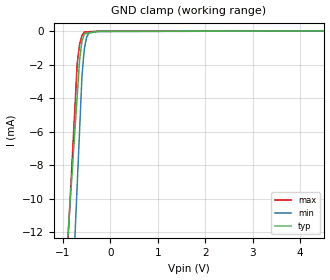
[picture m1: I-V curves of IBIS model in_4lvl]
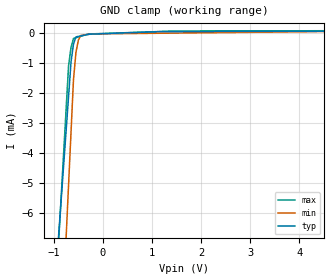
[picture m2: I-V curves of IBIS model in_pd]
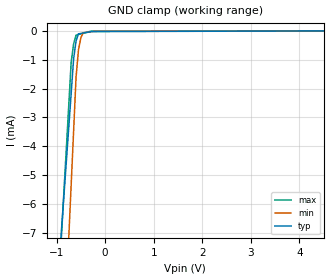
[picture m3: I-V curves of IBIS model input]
[IBIS Ver]   3.2
[Comment Char] |_char
[File Name]   pcm3168tpap.ibs
[File Rev]   3.0
[Source]
| This model file was created by Teraspeed Consulting Group LLC
| (http://www.teraspeed.com/).
[Date]   05-08-2008
[Notes]   Quality Check of this IBIS model: Model Passes IBIS Check
   Model parses into ICX IS. Simulation done with Hyperlynx.
   1. MIN TYP MAX information is based on Temprature and Voltage
   characteristics only.
[Disclaimer]
| This model is designed as an aid for customers of Texas Instruments.
| TI and its licensors and suppliers make no warranties, either expressed
| or implied, with respect to this  model, including the warranties of
| merchantability or fitness for a particular purpose.
| The model is provided solely on an "as is" basis. The entire risk as to
| its quality and performance is with the customer.
[Copyright]
| (C) Copyright 2008 Texas Instruments Incorporated. All rights reserved.
[Component]   PCM3168TPAP
[Manufacturer] TI
[Package]
| variable   typ   min   max
R_pkg  6.05E-02  5.80E-02  6.50E-02
L_pkg  5.05E-09  4.85E-09  5.38E-09
C_pkg  2.68E-13  2.40E-13  3.00E-13
[Pin] signal_name  model_name  R_pin  L_pin C_pin
1   VCOMAD   term   6.50E-02  5.38E-09  3.00E-13
2   AGNDAD2   GND   6.30E-02  5.25E-09  2.90E-13
3   VCCAAD2   POWER   6.20E-02  5.13E-09  2.80E-13
4   RST   in_pd   6.00E-02  5.04E-09  2.70E-13
5   OVF   output  5.90E-02  4.95E-09  2.60E-13
6   LRCKAD   io_pd   5.90E-02  4.90E-09  2.50E-13
7   BCKAD   io_pd   5.80E-02  4.87E-09  2.50E-13
8   DOUT1   output  5.80E-02  4.85E-09  2.40E-13
9   DOUT2   output  5.80E-02  4.85E-09  2.40E-13
10   DOUT3   output  5.80E-02  4.87E-09  2.50E-13
11   DGND2   GND   5.90E-02  4.90E-09  2.50E-13
12   VDD2   POWER   5.90E-02  4.95E-09  2.60E-13
13   ZERO   output  6.00E-02  5.04E-09  2.70E-13
14   VCCDA1   POWER   6.20E-02  5.13E-09  2.80E-13
15   VCOMDA   term   6.30E-02  5.25E-09  2.90E-13
16   AGNDDA1   GND   6.50E-02  5.38E-09  3.00E-13
17   VOUT8+   term   6.50E-02  5.38E-09  3.00E-13
18   VOUT8-   term   6.30E-02  5.25E-09  2.90E-13
19   VOUT7+   term   6.20E-02  5.13E-09  2.80E-13
20   VOUT7-   term   6.00E-02  5.04E-09  2.70E-13
21   VOUT6+   term   5.90E-02  4.95E-09  2.60E-13
22   VOUT6-   term   5.90E-02  4.90E-09  2.50E-13
23   VOUT5+   term   5.80E-02  4.87E-09  2.50E-13
24   VOUT5-   term   5.80E-02  4.85E-09  2.40E-13
25   VOUT4+   term   5.80E-02  4.85E-09  2.40E-13
26   VOUT4-   term   5.80E-02  4.87E-09  2.50E-13
27   VOUT3+   term   5.90E-02  4.90E-09  2.50E-13
28   VOUT3-   term   5.90E-02  4.95E-09  2.60E-13
29   VOUT2+   term   6.00E-02  5.04E-09  2.70E-13
30   VOUT2-   term   6.20E-02  5.13E-09  2.80E-13
31   VOUT1+   term   6.30E-02  5.25E-09  2.90E-13
32   VOUT1-   term   6.50E-02  5.38E-09  3.00E-13
33   AGNDDA2   GND   6.50E-02  5.38E-09  3.00E-13
34   VCCDA2   POWER   6.30E-02  5.25E-09  2.90E-13
35   LRCKDA   io_pd   6.20E-02  5.13E-09  2.80E-13
36   BCKDA   io_pd   6.00E-02  5.04E-09  2.70E-13
37   DIN1   input   5.90E-02  4.95E-09  2.60E-13
38   DIN2   input   5.90E-02  4.90E-09  2.50E-13
39   DIN3   input   5.80E-02  4.87E-09  2.50E-13
40   DIN4   input   5.80E-02  4.85E-09  2.40E-13
41   SCKI   input   5.80E-02  4.85E-09  2.40E-13
42   MC/SCL/FMT   input   5.80E-02  4.87E-09  2.50E-13
43   MDI/SDA/DEMP io_od   5.90E-02  4.90E-09  2.50E-13
44   MDO/ADR1/MD1 io   5.90E-02  4.95E-09  2.60E-13
45   MS/ADR0/MD0  in_pd   6.00E-02  5.04E-09  2.70E-13
46   VDD1   POWER   6.20E-02  5.13E-09  2.80E-13
47   DGND1   GND   6.30E-02  5.25E-09  2.90E-13
48   MODE   in_4lvl 6.50E-02  5.38E-09  3.00E-13
49   VCCAD1   POWER   6.50E-02  5.38E-09  3.00E-13
50   AGNDAD1   GND   6.30E-02  5.25E-09  2.90E-13
51   VIN1-   term   6.20E-02  5.13E-09  2.80E-13
52   VIN1+   term   6.00E-02  5.04E-09  2.70E-13
53   VIN2-   term   5.90E-02  4.95E-09  2.60E-13
54   VIN2+   term   5.90E-02  4.90E-09  2.50E-13
55   VIN3-   term   5.80E-02  4.87E-09  2.50E-13
56   VIN3+   term   5.80E-02  4.85E-09  2.40E-13
57   VIN4-   term   5.80E-02  4.85E-09  2.40E-13
58   VIN4+   term   5.80E-02  4.87E-09  2.50E-13
59   VREFAD1   term   5.90E-02  4.90E-09  2.50E-13
60   VREFAD2   term   5.90E-02  4.95E-09  2.60E-13
61   VIN5-   term   6.00E-02  5.04E-09  2.70E-13
62   VIN5+   term   6.20E-02  5.13E-09  2.80E-13
63   VIN6-   term   6.30E-02  5.25E-09  2.90E-13
64   VIN6+   term   6.50E-02  5.38E-09  3.00E-13
[Diff Pin] inv_pin vdiff tdelay_typ tdelay_min tdelay_max
17   18   NA   NA   NA   NA
19   20   NA   NA   NA   NA
21   22   NA   NA   NA   NA
23   24   NA   NA   NA   NA
25   26   NA   NA   NA   NA
27   28   NA   NA   NA   NA
29   30   NA   NA   NA   NA
31   32   NA   NA   NA   NA
52   51   NA   NA   NA   NA
54   53   NA   NA   NA   NA
56   55   NA   NA   NA   NA
58   57   NA   NA   NA   NA
62   61   NA   NA   NA   NA
64   63   NA   NA   NA   NA
[Model] term
Model_type Terminator
C_comp   0  0  0
| variable   typ   min   max
[Voltage Range]   5.00000V  4.75000V  5.25000V
[POWER Clamp Reference]  5.00000V  4.75000V  5.25000V
[GND Clamp Reference]   0.00000V  0.00000V  0.00000V
[Temperature Range]   25   105   -40
| Models and submodels in the file (8): term (Terminator), in_4lvl (Input), in_pd (Input), input (Input), io (I/O), io_od (I/O_open_drain), io_pd (I/O), output (Output)
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[Model] in_4lvl
Model_type Input
Vinl = 800.000mV
Vinh = 2.00000V
C_comp 714.000fF 714.000fF 714.000fF
| variable typ   min   max
[Voltage Range] 3.30000V 3.00000V 3.60000V
[POWER Clamp Reference] 3.30000V 3.00000V 3.60000V
[GND Clamp Reference] 0.00000V 0.00000V 0.00000V
[Temperature Range]   25   105   -40
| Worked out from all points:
|   GND clamp passes 1 mA (typ) near -0.62 V on its own axis
[GND Clamp]
-3.3V     -114.6mA   -177.2mA   -143mA
-700mV    -3.834mA   -9.148mA   -1.914mA
-650mV    -1.704mA   -5.915mA   -791.6uA
-600mV    -601.6uA   -2.683mA   -258.2uA
-550mV    -171.1uA   -1.063mA   -66.76uA
-500mV    -146.9uA   -356.5uA   -56.99uA
-450mV    -122.7uA   -95.27uA   -47.22uA
-275mV    -37.99uA   -37.18uA   -13.04uA
-225mV    -37.54uA   -20.58uA   -12.88uA
6.6V      22.81uA    16.82uA    8.375uA
[POWER Clamp]
-3.3V     0A         0A         0A
6.6V      0A         0A         0A
[Model] in_pd
Model_type Input
Vinl = 800.000mV
Vinh = 2.00000V
C_comp 739.000fF 739.000fF 739.000fF
| variable typ   min   max
[Voltage Range] 3.30000V 3.00000V 3.60000V
[POWER Clamp Reference] 3.30000V 3.00000V 3.60000V
[GND Clamp Reference] 0.00000V 0.00000V 0.00000V
[Temperature Range]   25   105   -40
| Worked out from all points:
|   GND clamp passes 1 mA (typ) near -0.65 V on its own axis
[GND Clamp]
-3.3V     -61.68mA   -96.51mA   -76.65mA
-700mV    -2.122mA   -5.079mA   -1.097mA
-650mV    -976.7uA   -3.32mA    -481.8uA
-600mV    -370.7uA   -1.562mA   -183.4uA
-550mV    -128.6uA   -650uA     -158.2uA
-500mV    -112.3uA   -238.5uA   -133uA
-450mV    -96.05uA   -80.53uA   -107.8uA
-300mV    -47.29uA   -47.16uA   -32.22uA
-225mV    -36.17uA   -30.47uA   -27.99uA
1.45V     50.09uA    -2.108uA   66.54uA
6.6V      68.46uA    85.1uA     83.9uA
[POWER Clamp]
-3.3V     0A         0A         0A
6.6V      0A         0A         0A
[Model] input
Model_type Input
Vinl = 800.000mV
Vinh = 2.00000V
C_comp 538.000fF 538.000fF 538.000fF
| variable typ   min   max
[Voltage Range] 3.30000V 3.00000V 3.60000V
[POWER Clamp Reference] 3.30000V 3.00000V 3.60000V
[GND Clamp Reference] 0.00000V 0.00000V 0.00000V
[Temperature Range]   25   105   -40
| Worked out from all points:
|   GND clamp passes 1 mA (typ) near -0.65 V on its own axis
[GND Clamp]
-3.3V     -63.83mA   -101.9mA   -79.25mA
-700mV    -2.156mA   -5.322mA   -1.079mA
-650mV    -970.2uA   -3.465mA   -451.1uA
-600mV    -347.4uA   -1.607mA   -147.9uA
-550mV    -99.42uA   -655.3uA   -124.6uA
-500mV    -85.4uA    -227.4uA   -101.2uA
-450mV    -71.38uA   -63.1uA    -77.89uA
-300mV    -29.31uA   -30.65uA   -7.836uA
-275mV    -22.3uA    -25.24uA   -7.789uA
-225mV    -22.04uA   -14.43uA   -7.694uA
6.6V      13.26uA    11.26uA    5.18uA
[POWER Clamp]
-3.3V     0A         0A         0A
6.6V      0A         0A         0A
